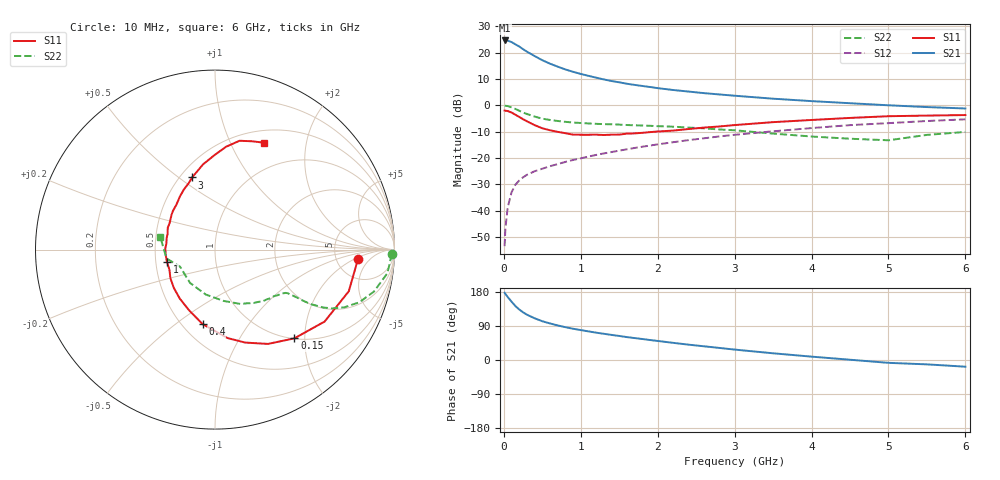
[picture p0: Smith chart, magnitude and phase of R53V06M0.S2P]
! SIEMENS Small Signal Semiconductors
! BFR183
! Si NPN RF Bipolar Junction Transistor in SOT23
! VCE = 3 V  IC = 6 mA
! Common Emitter S-Parameters:  May  1996
# GHz  S  MA  R  50
!  f  S11  S21  S12  S22
! GHz  MAG  ANG  MAG  ANG  MAG  ANG  MAG  ANG
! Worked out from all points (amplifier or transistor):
!   36 points, 10 MHz to 6 GHz, reference 50 ohm
!   highest |S21| = 24.7 dB at 10 MHz (marker M1)
!   |S21| within 3 dB of that: start of sweep to 234.4 MHz
!   unconditionally stable (mu >= 1): 947.7 MHz to 2.588 GHz
!   at 250 MHz: K = 0.47, MSG = 24.4 dB, |S12| = -27.4 dB
!   at 1.4 GHz: K = 1.06, MAG = 12.0 dB, |S12| = -17.8 dB
!   at 6 GHz: K = 0.89, MSG = 2.1 dB, |S12| = -5.3 dB
!   lowest NFmin = 1.20 dB at 450 MHz
!   S11 on the Smith chart (normalised r, x): 10 MHz: 8.21, -2.25; 150 MHz: 1.01, -1.78; 400 MHz: 0.63, -0.63; 1 GHz: 0.57, -0.08; 3 GHz: 0.57, +0.56; 6 GHz: 0.64, +1.34
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0.01  0.7966 -3.6  17.15 177.4  0.0021 86.5  0.9875 -1.5
0.02  0.7905 -6.9  16.98 174.4  0.0045 86.3  0.9802 -3.1
0.05  0.7807 -17.3  16.98 166.4  0.0114 81.5  0.9694 -7.8
0.1  0.7305 -33.3  15.97 154.0  0.0222 74.6  0.9159 -14.8
0.15  0.6633 -48.2  14.48 142.3  0.031 68.3  0.8554 -20.1
0.2  0.6026 -60.7  13.15 133.3  0.0372 63.9  0.7899 -24.0
0.25  0.5447 -72.0  11.7 125.8  0.0428 60.6  0.7315 -26.6
0.3  0.4979 -81.9  10.49 119.6  0.0478 59.1  0.6855 -28.1
0.4  0.4206 -99.5  8.659 110.1  0.0558 57.3  0.6117 -29.7
0.5  0.3663 -113.6  7.22 102.3  0.0624 57.5  0.5585 -30.2
0.6  0.336 -125.8  6.209 96.5  0.0696 57.7  0.5275 -30.3
0.8  0.2954 -147.2  4.814 86.6  0.084 58.8  0.4862 -30.8
1  0.2762 -166.0  3.957 78.9  0.0983 60.2  0.4617 -31.5
1.1  0.2761 -173.5  3.64 75.5  0.1062 60.6  0.4529 -32.5
1.3  0.2729 173.0  3.11 69.2  0.122 60.6  0.4396 -34.0
1.6  0.2898 155.3  2.576 60.4  0.1459 60.1  0.4228 -37.5
2.2  0.3309 130.3  1.96 45.3  0.1991 57.4  0.393 -46.8
3  0.4218 107.6  1.525 27.5  0.2754 50.4  0.3357 -64.6
3.5  0.4794 98.0  1.339 17.7  0.3212 44.7  0.2903 -80.3
4.5  0.5768 83.8  1.098 0.7  0.4206 32.7  0.232 -126.8
5.5  0.6388 70.8  0.928 -11.5  0.5041 20.4  0.2743 -169.6
6  0.6542 65.6  0.872 -17.7  0.5424 12.4  0.3127 167.1
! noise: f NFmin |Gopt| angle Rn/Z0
0.45  1.2  0.21  41  0.24
0.9  1.25  0.24  101  0.21
1.8  2  0.32  175  0.14
